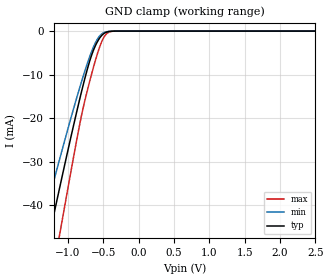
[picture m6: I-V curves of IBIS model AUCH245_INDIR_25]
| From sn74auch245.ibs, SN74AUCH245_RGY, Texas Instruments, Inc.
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[Model]   AUCH245_INDIR_25
Model_type  Input
Vinl=0.7
Vinh=1.7
| variable   typ   min   max
C_comp   2.47pF   1.97pF   2.90pF
[Temperature Range]   40   100   -40
| Ambient temperature   25   85   -40
[Voltage range]   2.5   2.3   2.7
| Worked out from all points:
|   GND clamp passes 1 mA (typ) near -0.52 V on its own axis
[GND Clamp]
| AUCH245_INDIR_25
|   Voltage   I(typ)   I(min)   I(max)
-3.6V     -229.3mA   -192.6mA   -273mA
-1.38V    -55.83mA   -45.62mA   -70.82mA
-1.28V    -48.21mA   -39.37mA   -61.64mA
-1.235V   -44.81mA   -36.59mA   -57.52mA
-1.11V    -35.45mA   -28.97mA   -46.07mA
-830mV    -15.39mA   -12.79mA   -21.13mA
-710mV    -7.848mA   -6.681mA   -12.62mA
-600mV    -2.951mA   -2.314mA   -6.078mA
-490mV    -542.1uA   -342.5uA   -1.378mA
-430mV    -133.4uA   -89.21uA   -324.3uA
-340mV    -10.37uA   -9.319uA   -15.22uA
2.5V      453pA      1.243nA    77.67pA
